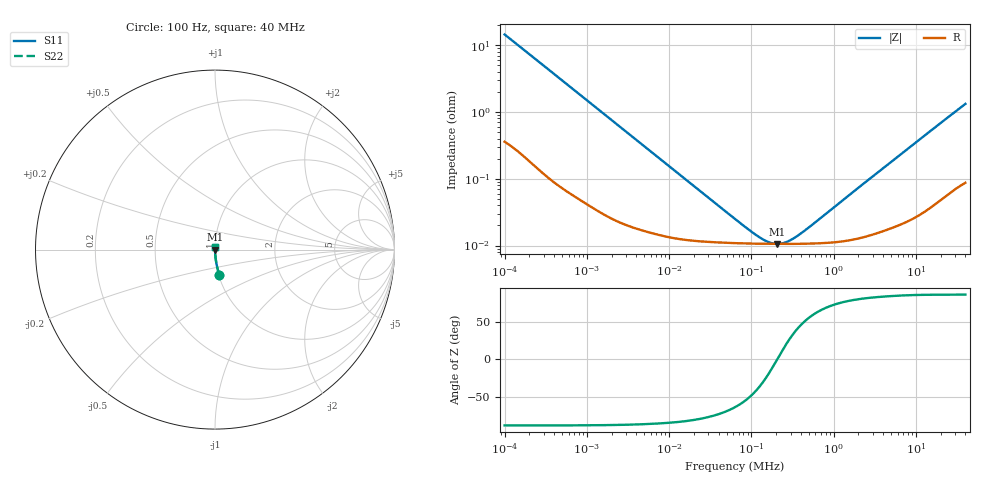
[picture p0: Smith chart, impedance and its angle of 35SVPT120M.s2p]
!  *** S-Parameter ***
!  Copyright (C) Panasonic Industry
!  Conductive Polymer Aluminum Solid Capacitors (OS-CON)
!  Parts No. 35SVPT120M
! Touchstone file from project
# GHZ S RI R 50.000000
! Modal data exported
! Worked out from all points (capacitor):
!   450 points, 100 Hz to 40 MHz, reference 50 ohm
!   read as one part in series: C = 109 uF near 105.9 Hz
!   lowest |Z| = 10.6 mohm at 205.4 kHz (marker M1)
!   series resonance near 207 kHz, so ESL is about 5.4 nH
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1e-07  0.0238 -0.1406  0.9762 0.1406  0.9762 0.1406  0.0238 -0.1406
1.059254e-07  0.0216 -0.1332  0.9784 0.1332  0.9784 0.1332  0.0216 -0.1332
1.584893e-07  0.0107 -0.0909  0.9893 0.0909  0.9893 0.0909  0.0107 -0.0909
2.511886e-07  0.00482 -0.0582  0.9952 0.0582  0.9952 0.0582  0.00482 -0.0582
4.340103e-07  0.00198 -0.034  0.998 0.034  0.998 0.034  0.00198 -0.034
8.659643e-07  0.000761 -0.0172  0.9992 0.0172  0.9992 0.0172  0.000761 -0.0172
7.498942e-06  0.000148 -0.00205  0.9999 0.00205  0.9999 0.00205  0.000148 -0.00205
6.493816e-05  0.000109 -0.000218  0.9999 0.000218  0.9999 0.000218  0.000109 -0.000218
0.0001  0.000107 -0.000121  0.9999 0.000121  0.9999 0.000121  0.000107 -0.000121
0.0001333521  0.000106 -6.94e-05  0.9999 6.94e-05  0.9999 6.94e-05  0.000106 -6.94e-05
0.0001496236  0.000106 -5.05e-05  0.9999 5.05e-05  0.9999 5.05e-05  0.000106 -5.05e-05
0.0001678804  0.000106 -3.23e-05  0.9999 3.23e-05  0.9999 3.23e-05  0.000106 -3.23e-05
0.0001883649  0.000106 -1.45e-05  0.9999 1.45e-05  0.9999 1.45e-05  0.000106 -1.45e-05
0.0002053525  0.000106 -1.22e-06  0.9999 1.22e-06  0.9999 1.22e-06  0.000106 -1.22e-06
0.0002440619  0.000106 2.54e-05  0.9999 -2.54e-05  0.9999 -2.54e-05  0.000106 2.54e-05
0.0002985383  0.000106 5.74e-05  0.9999 -5.74e-05  0.9999 -5.74e-05  0.000106 5.74e-05
0.0003868121  0.000106 0.000102  0.9999 -0.000102  0.9999 -0.000102  0.000106 0.000102
0.0005463865  0.000107 0.000173  0.9999 -0.000173  0.9999 -0.000173  0.000107 0.000173
0.001830206  0.000125 0.000661  0.9999 -0.000661  0.9999 -0.000661  0.000125 0.000661
0.004731513  0.00018 0.00168  0.9998 -0.00168  0.9998 -0.00168  0.00018 0.00168
0.01938653  0.000509 0.00661  0.9995 -0.00661  0.9995 -0.00661  0.000509 0.00661
0.04  0.00104 0.0132  0.999 -0.0132  0.999 -0.0132  0.00104 0.0132
